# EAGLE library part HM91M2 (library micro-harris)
MICROCONTROLLER/MEMORY DEVICE
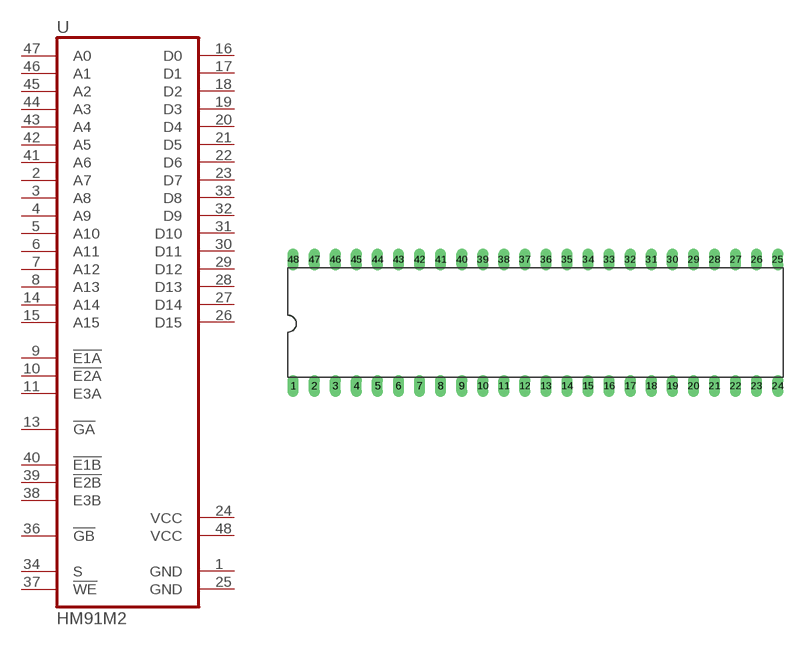
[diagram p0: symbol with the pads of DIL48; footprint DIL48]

Designator prefix U

## HM91M2 (OC_FARNELL: unknown; OC_NEWARK: unknown)  [DIL48]
1  GND  pwr
2  A7  in
3  A8  in
4  A9  in
5  A10  in
6  A11  in
7  A12  in
8  A13  in
9  !E1A  in
10  !E2A  in
11  E3A  in
13  !GA  in
14  A14  in
15  A15  in
16  D0
17  D1
18  D2
19  D3
20  D4
21  D5
22  D6
23  D7
24  VCC  pwr
25  GND  pwr
26  D15
27  D14
28  D13
29  D12
30  D11
31  D10
32  D9
33  D8
34  S  in
36  !GB  in
37  !WE  in
38  E3B  in
39  !E2B  in
40  !E1B  in
41  A6  in
42  A5  in
43  A4  in
44  A3  in
45  A2  in
46  A1  in
47  A0  in
48  VCC  pwr

## Footprint DIL48 (pad centres in mm)
Dual In Line Package
drill 0.813 long: 1 -29.21,-7.62; 2 -26.67,-7.62; 3 -24.13,-7.62; 4 -21.59,-7.62; 5 -19.05,-7.62; 6 -16.51,-7.62; 7 -13.97,-7.62; 8 -11.43,-7.62; 9 -8.89,-7.62; 10 -6.35,-7.62; 11 -3.81,-7.62; 12 -1.27,-7.62; 13 1.27,-7.62; 14 3.81,-7.62; 15 6.35,-7.62; 16 8.89,-7.62; 17 11.43,-7.62; 18 13.97,-7.62; 19 16.51,-7.62; 20 19.05,-7.62; 21 21.59,-7.62; 22 24.13,-7.62; 23 26.67,-7.62; 24 29.21,-7.62; 25 29.21,7.62; 26 26.67,7.62; 27 24.13,7.62; 28 21.59,7.62; 29 19.05,7.62; 30 16.51,7.62; 31 13.97,7.62; 32 11.43,7.62; 33 8.89,7.62; 34 6.35,7.62; 35 3.81,7.62; 36 1.27,7.62; 37 -1.27,7.62; 38 -3.81,7.62; 39 -6.35,7.62; 40 -8.89,7.62; 41 -11.43,7.62; 42 -13.97,7.62; 43 -16.51,7.62; 44 -19.05,7.62; 45 -21.59,7.62; 46 -24.13,7.62; 47 -26.67,7.62; 48 -29.21,7.62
